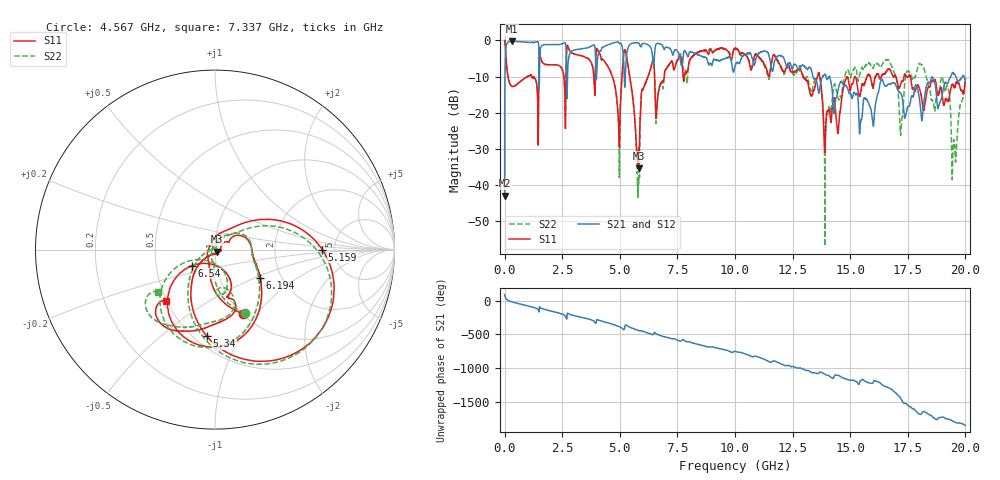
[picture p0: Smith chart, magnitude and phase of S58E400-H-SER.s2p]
!{S58E400}
!Johanson Technology Inc.
!www.johansontechnology.com
!Test Board Conditions:
!Substrate Type  RO4350B
!Substrate Thickness  60 mil
!Substrate Dk  3.66
!TL Type: GCPW
!TL Trace Width  115 mil
!TL Gap  52 mil
!Electrode orientation  Horizontal
!DUT TOPOLOGY	SERIES
!Mounting Pad LxW  55x428 mil
! Created Wed Apr 14 11:47:47 2021
# mhz S ma R 50
! 2 Port Network Data from SP1.SP block
! freq  magS11  angS11  magS21  angS21  magS12  angS12  magS22  angS22
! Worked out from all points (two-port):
!   20001 points, 300 kHz to 20 GHz, reference 50 ohm
!   highest |S21| = -0.25 dB at 336.3 MHz (marker M1); lowest = -42.9 dB at 300 kHz (marker M2)
!   |S21| within 3 dB of the highest: 40.23 MHz to 1.486 GHz (1.446 GHz wide, 189 % of centre); 1.535 GHz to 2.673 GHz (1.138 GHz wide, 54.1 % of centre)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
!   lowest |S11| = -35.3 dB at 5.818 GHz (marker M3), VSWR 1.04, Z = 51.2 - j1.24 ohm
!   |S11| at or under -10 dB: 146.8 MHz to 979.9 MHz (833.1 MHz wide, 148 % of centre); 13.68 GHz to 15.21 GHz (1.524 GHz wide, 10.5 % of centre); 17.61 GHz to end of sweep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
!   |S22| runs from -56.8 to 0.0 dB; largest |S21 - S12| = 0.01
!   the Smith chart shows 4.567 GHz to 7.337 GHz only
!   S11 on the Smith chart (normalised r, x): 4.567 GHz: 1.01, -0.85; 5.159 GHz: 3.97, +0.00; 5.34 GHz: 0.58, -0.73; 6.194 GHz: 1.56, -0.55; 6.54 GHz: 0.76, -0.14; 7.337 GHz: 0.50, -0.34
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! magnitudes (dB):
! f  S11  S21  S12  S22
! 300 kHz  0.0  -42.9  -42.8  0.0
! 108.3 MHz  -8.2  -0.7  -0.7  -8.2
! 336.3 MHz  -12.7  -0.3  -0.3  -12.7
! 3.334 GHz  -4.2  -2.3  -2.3  -4.2
! 4.567 GHz  -8.2  -1.0  -1.0  -8.2
! 4.951 GHz  -23.2  -0.6  -0.6  -23.3
! 5.159 GHz  -4.5  -5.0  -5.0  -4.4
! 5.34 GHz  -6.3  -2.4  -2.4  -6.4
! 5.818 GHz  -35.3  -0.7  -0.7  -38.2
! 6.194 GHz  -10.5  -1.1  -1.1  -10.5
! 6.54 GHz  -16.0  -1.7  -1.7  -16.1
! 6.667 GHz  -14.6  -0.8  -0.8  -14.8
! 7.337 GHz  -8.1  -3.5  -3.5  -8.0
! 10 GHz  -2.2  -7.1  -7.1  -2.2
! 13.33 GHz  -15.2  -8.5  -8.5  -14.3
! 13.93 GHz  -25.9  -9.5  -9.4  -26.5
! 16.67 GHz  -7.8  -12.0  -12.1  -5.5
! 17.21 GHz  -11.8  -14.8  -14.8  -24.4
! 17.5 GHz  -10.0  -18.3  -18.3  -8.5
! 19.01 GHz  -16.0  -14.5  -14.4  -10.5
! 19.5 GHz  -12.9  -9.2  -9.1  -27.6
! 20 GHz  -10.6  -11.5  -11.5  -11.8
